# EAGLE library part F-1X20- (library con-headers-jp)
FEMALE HEADER
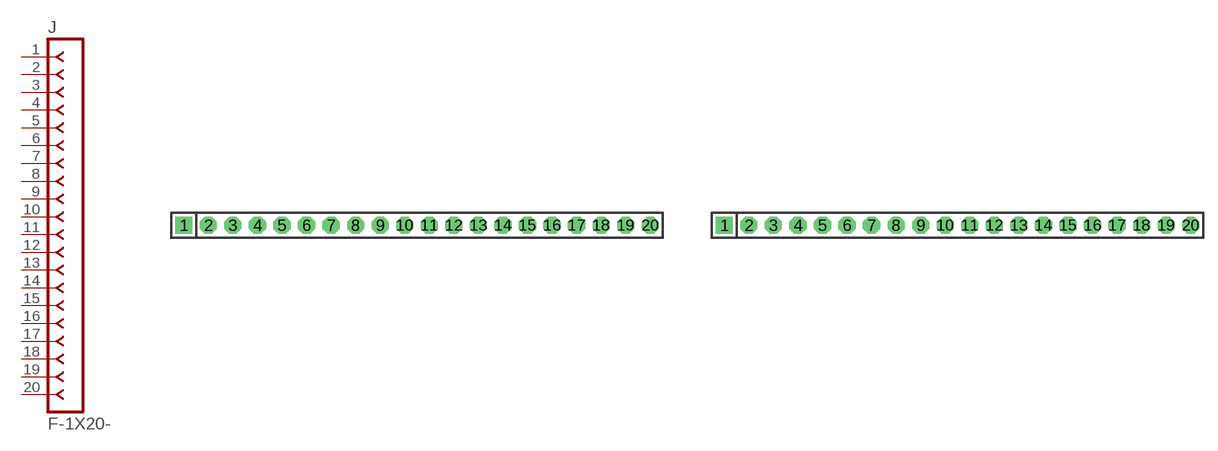
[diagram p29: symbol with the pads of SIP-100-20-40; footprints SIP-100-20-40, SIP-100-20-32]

Designator prefix J

## F-1X20-SIP-100-40  [SIP-100-20-40]
1  1  pas
2  2  pas
3  3  pas
4  4  pas
5  5  pas
6  6  pas
7  7  pas
8  8  pas
9  9  pas
10  10  pas
11  11  pas
12  12  pas
13  13  pas
14  14  pas
15  15  pas
16  16  pas
17  17  pas
18  18  pas
19  19  pas
20  20  pas

## F-1X20-SIP-100-32  [SIP-100-20-32]
Pads as for SIP-100-20-40

## F-1X20-SIP-100-32Y  [SIP-100-20-32Y]
Pads as for SIP-100-20-40

## F-1X20-SIP-100-40Y  [SIP-100-20-40Y]
Pads as for SIP-100-20-40

## F-1X20-KK-4455-B20  [KK-4455-B20]
Pads as for SIP-100-20-40

## F-1X20-KK-4455-C20  [KK-4455-C20]
Pads as for SIP-100-20-40

## F-1X20-KK-4455-A20  [KK-4455-A20]
Pads as for SIP-100-20-40

## Footprint SIP-100-20-40 (pad centres in mm)
SIP Header - 0.1", 40 mil drill
drill 1.016 pad 1.778 square: 1 -24.13,0
drill 1.016 pad 1.778 octagon: 2 -21.59,0; 3 -19.05,0; 4 -16.51,0; 5 -13.97,0; 6 -11.43,0; 7 -8.89,0; 8 -6.35,0; 9 -3.81,0; 10 -1.27,0; 11 1.27,0; 12 3.81,0; 13 6.35,0; 14 8.89,0; 15 11.43,0; 16 13.97,0; 17 16.51,0; 18 19.05,0; 19 21.59,0; 20 24.13,0

## Footprint SIP-100-20-32 (pad centres in mm)
SIP Header - 0.1", 32 mil drill
drill 0.813 pad 1.778 square: 1 -24.13,0
drill 0.813 pad 1.778 octagon: 2 -21.59,0; 3 -19.05,0; 4 -16.51,0; 5 -13.97,0; 6 -11.43,0; 7 -8.89,0; 8 -6.35,0; 9 -3.81,0; 10 -1.27,0; 11 1.27,0; 12 3.81,0; 13 6.35,0; 14 8.89,0; 15 11.43,0; 16 13.97,0; 17 16.51,0; 18 19.05,0; 19 21.59,0; 20 24.13,0

## Footprint SIP-100-20-32Y (pad centres in mm)
SIP Header - 0.1", 32 mil drill
drill 0.813 long: 1 -24.13,0; 2 -21.59,0; 3 -19.05,0; 4 -16.51,0; 5 -13.97,0; 6 -11.43,0; 7 -8.89,0; 8 -6.35,0; 9 -3.81,0; 10 -1.27,0; 11 1.27,0; 12 3.81,0; 13 6.35,0; 14 8.89,0; 15 11.43,0; 16 13.97,0; 17 16.51,0; 18 19.05,0; 19 21.59,0; 20 24.13,0

## Footprint SIP-100-20-40Y (pad centres in mm)
SIP Header - 0.1", 40 mil drill
drill 1.016 long: 1 -24.13,0; 2 -21.59,0; 3 -19.05,0; 4 -16.51,0; 5 -13.97,0; 6 -11.43,0; 7 -8.89,0; 8 -6.35,0; 9 -3.81,0; 10 -1.27,0; 11 1.27,0; 12 3.81,0; 13 6.35,0; 14 8.89,0; 15 11.43,0; 16 13.97,0; 17 16.51,0; 18 19.05,0; 19 21.59,0; 20 24.13,0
